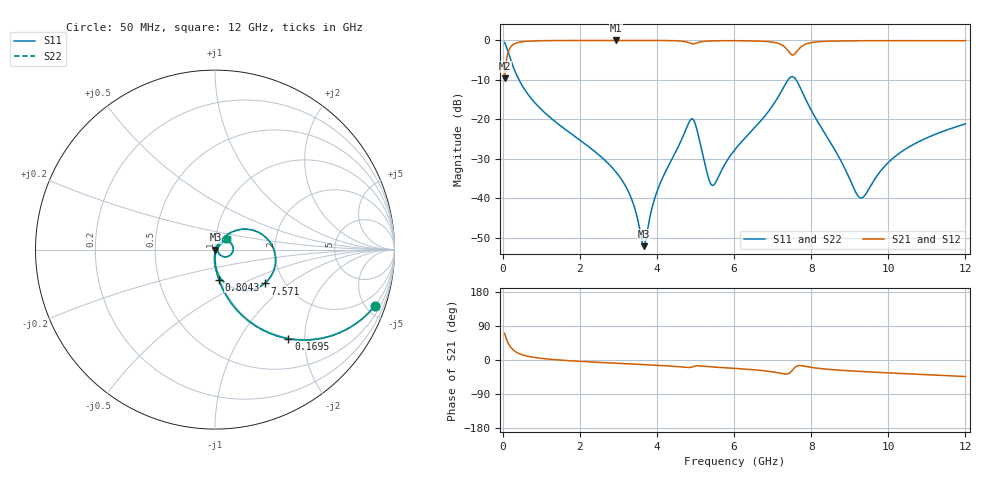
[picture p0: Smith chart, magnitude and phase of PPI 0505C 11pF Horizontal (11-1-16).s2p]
# MHz S MA R 50
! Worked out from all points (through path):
!   1601 points, 50 MHz to 12 GHz, reference 50 ohm
!   highest |S21| = -0.02 dB at 2.948 GHz (marker M1); lowest = -9.6 dB at 50 MHz (marker M2)
!   group delay of S21, straight-line fit = 12.3 ps
!   lowest |S11| = -52.2 dB at 3.657 GHz (marker M3), VSWR 1.00, Z = 50.2 - j0.064 ohm
!   |S11| at or under -10 dB: 423.5 MHz to 7.4 GHz (6.977 GHz wide, 178 % of centre); 7.61 GHz to end of sweep
!   |S22| runs from -52.2 to -0.5 dB; largest |S21 - S12| = 0
!   S11 on the Smith chart (normalised r, x): 50 MHz: 0.98, -5.66; 169.5 MHz: 0.98, -1.67; 804.3 MHz: 0.99, -0.34; 7.571 GHz: 1.59, -0.67; 12 GHz: 1.13, +0.13
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50  0.9436 -19.5  0.3308 70.5  0.3308 70.5  0.9436 -19.5
169.5  0.6431 -50.5  0.7654 39.5  0.7654 39.5  0.6431 -50.5
371.1562  0.3562 -70.3  0.9338 19.6  0.9338 19.6  0.3562 -70.3
804.3438  0.1685 -82.7  0.9847 7.0  0.9847 7.0  0.1685 -82.7
2044.156  0.05265 -92.3  0.9971 -3.8  0.9971 -3.8  0.05265 -92.3
2947.875  0.02117 -93.7  0.9978 -8.6  0.9978 -8.6  0.02117 -93.7
3336.25  0.009967 -88.5  0.9977 -10.5  0.9977 -10.5  0.009967 -88.5
3657.406  0.002468 -15.0  0.9973 -12.2  0.9973 -12.2  0.002468 -15.0
4038.312  0.01354 60.7  0.9961 -14.2  0.9961 -14.2  0.01354 60.7
4889.75  0.1007 10.2  0.9106 -19.0  0.9106 -19.0  0.1007 10.2
5009.25  0.08284 -26.7  0.9182 -15.7  0.9182 -15.7  0.08284 -26.7
5315.469  0.0197 -32.9  0.9807 -17.3  0.9807 -17.3  0.0197 -32.9
5427.5  0.01461 -2.5  0.9856 -18.2  0.9856 -18.2  0.01461 -2.5
6025  0.0414 55.6  0.99 -22.2  0.99 -22.2  0.0414 55.6
7234.938  0.2293 28.8  0.8791 -35.7  0.8791 -35.7  0.2293 28.8
7444.062  0.3354 -4.1  0.6948 -34.1  0.6948 -34.1  0.3354 -4.1
7571.031  0.3345 -34.3  0.6718 -20.1  0.6718 -20.1  0.3345 -34.3
7780.156  0.2162 -69.2  0.8564 -15.5  0.8564 -15.5  0.2162 -69.2
8019.156  0.1258 -85.0  0.9404 -19.7  0.9404 -19.7  0.1258 -85.0
9251.5  0.01025 -34.0  0.9892 -30.1  0.9892 -30.1  0.01025 -34.0
10013.31  0.02873 40.4  0.9913 -34.1  0.9913 -34.1  0.02873 40.4
12000  0.08747 42.4  0.9892 -43.5  0.9892 -43.5  0.08747 42.4
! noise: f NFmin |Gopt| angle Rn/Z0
50  0.0004048  0.874  1.71  0.0006931
1372  0.004038  0.6778  4.99  0.002417
2701  0.006832  0.6354  9.173  0.003507
4031  0.01195  0.6817  13.33  0.007175
5360  0.02978  0.8175  17.73  0.03334
6682  0.0335  0.8012  21.87  0.03369
8012  0.06624  0.8756  26.3  0.1091
9341  0.0299  0.7101  30.39  0.01895
1.067e+04  0.02673  0.6474  34.22  0.01319
1.2e+04  0.02709  0.6201  37.91  0.01198
